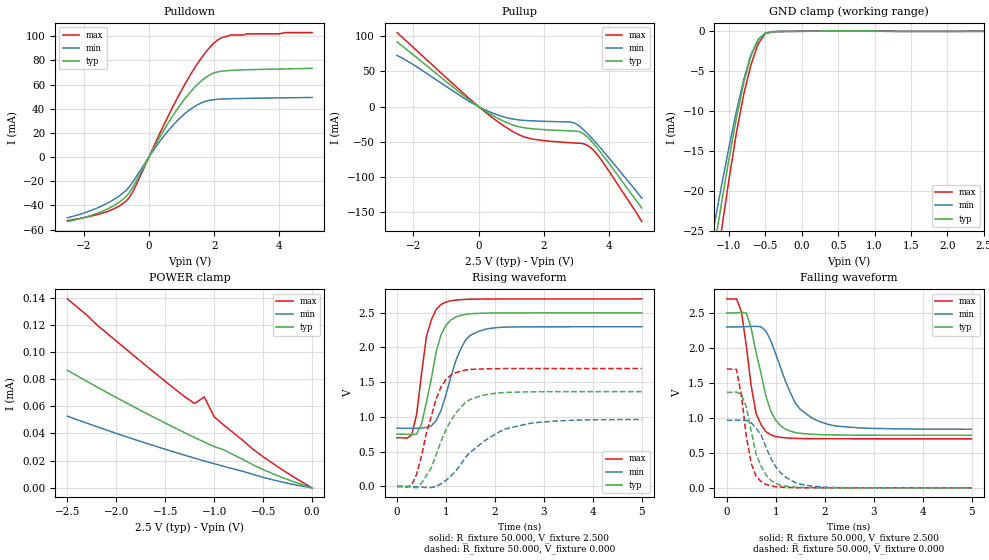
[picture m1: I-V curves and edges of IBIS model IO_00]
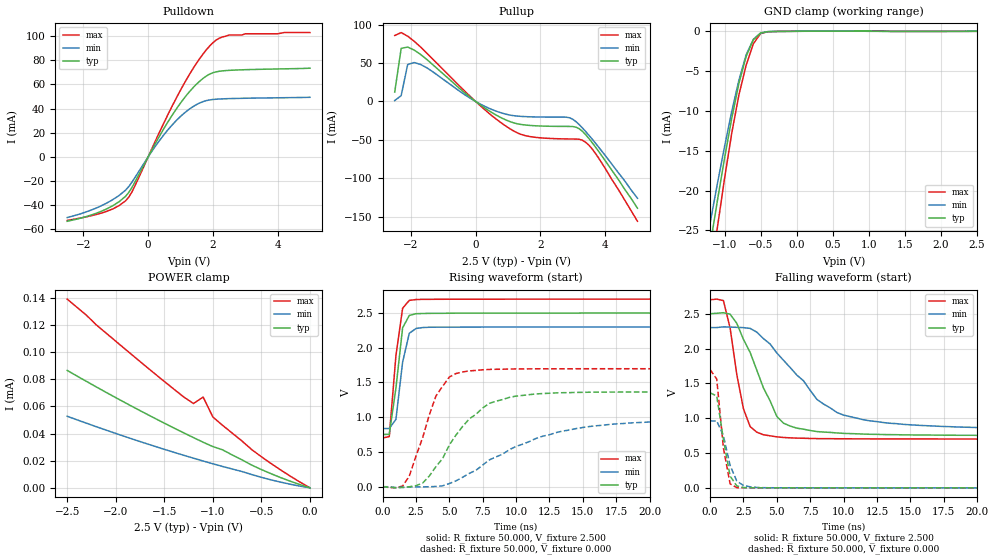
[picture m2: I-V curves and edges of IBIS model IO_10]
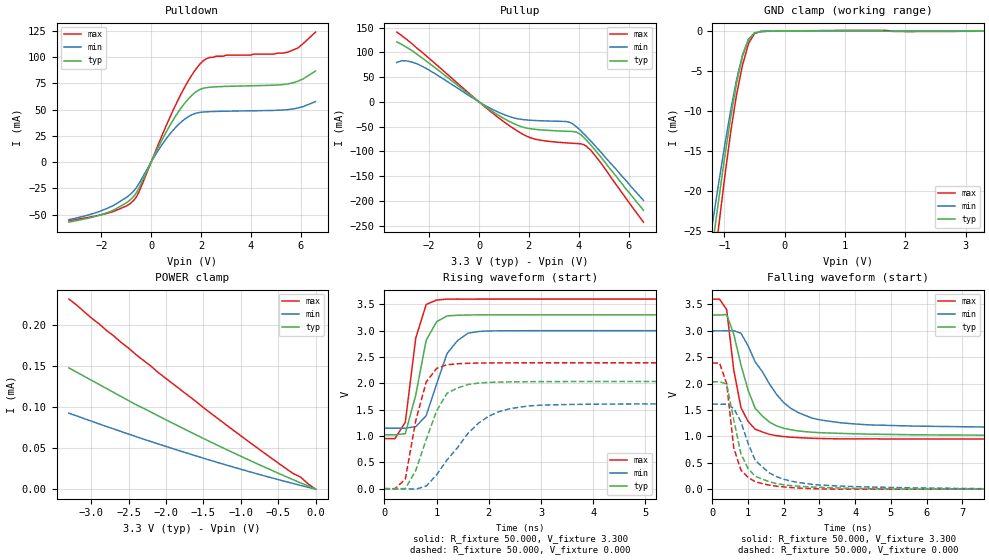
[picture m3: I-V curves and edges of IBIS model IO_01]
| / 7\'7   Xilinx XC9500XL I/O Buffer IBIS File
| \ \   Xilinx Inc.
| / /   2100 Logic Drive
| \_\/.\   San Jose,   CA 95124
[IBIS ver]   3.2
[File name]   trigger_a.ibs
[File Rev]   2.2
[Date]   Sat Aug 03 14:31:19 2002
[Source]   Spice netlist
[Notes]   - max/min process data included in this ibis model
   - Control flag setting:
   SLW=0 - fast slew rate
   SLW=1 - slow slew rate
   VIO=0 - 2.5V Vddio
   VIO=1 - 3.3V Vddio
   - Created by Joey Jia x4437
[Disclaimer] The data in this model is derived from SPICE simulations
   using modeling information extracted from the target pro-
   cess. While a great deal of care has been take to provide
   information that is accurate, this model is considered
   preliminary as it has not been verified by actual silicon
   measurement. Treat the data in this model as preliminary
   until actual silicon verification is performed.
[Copyright]   Xilinx Inc.
|   Component XC9500XL
|   >>> Make Your Selection of the Package type Below <<<
[Component]   XC9500XL
[Manufacturer]   Xilinx Inc.
[Package]
| variable   min   typ   max
R_pkg   0.079200   0.084800   0.090400
L_pkg   4.700nH   5.200nH   5.700nH
C_pkg   0.400pF   0.550pF   0.700pF
[Pin]  signal_name   model_name   R_pin   L_pin   C_pin
90   data<6>   IO_11
79   data<4>   IO_11
27   data<0>   IO_11
59   data<2>   IO_11
22   clock   IO_11
12   rd   IO_11
8   ctr_a1   IO_11
56   ctr_a0   IO_11
95   data<7>   IO_11
74   data<5>   IO_11
30   wr2   IO_11
99   wr0   IO_11
42   wr1   IO_11
91   ctr_data<3>   IO_11
85   ctr_data<5>   IO_11
92   ctr_data<7>   IO_11
1   ctr_data<1>   IO_11
23   ctr_data<2>   IO_11
3   ctr_data<4>   IO_11
77   ctr_data<6>   IO_11
94   data<3>   IO_11
89   ctr_data<0>   IO_11
18   data<1>   IO_11
13   addr<0>   IO_01
41   addr<10>   IO_01
87   addr<11>   IO_01
93   addr<12>   IO_01
96   addr<13>   IO_01
97   addr<14>   IO_01
14   addr<1>   IO_01
50   addr<2>   IO_01
53   addr<3>   IO_01
65   addr<4>   IO_01
37   addr<5>   IO_01
60   addr<6>   IO_01
61   addr<7>   IO_01
55   addr<8>   IO_01
64   addr<9>   IO_01
6   addr<15>   IO_01
28   clkout   IO_01
39   memrd   IO_01
11   ctlout<0>   IO_01
72   ctlout<1>   IO_01
76   ctlout<2>   IO_01
70   ctlout<3>   IO_01
86   ctlout<4>   IO_01
78   ctlout<5>   IO_01
82   ctlout<6>   IO_01
81   ctlout<7>   IO_01
10   go_out   IO_01
| Models and submodels in the file (4): IO_00 (I/O), IO_10 (I/O), IO_01 (I/O), IO_11 (I/O)
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|   Model IO_00
[Model]   IO_00
Model_type   I/O
Polarity   Inverting
Enable   Active-High
Vinl =   0.800V
Vinh =   2.000V
Vmeas =   1.250V
Cref =  50.000pF
Rref =   1.000M
Vref =  0.000V
C_comp   6.700pF   5.700pF   7.600pF
[Temperature Range]   50.000   100.000   0.000
[Voltage Range]   2.500V   2.300V   2.700V
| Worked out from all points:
|   slope of the pulldown table from 0 to 0.375 V, typ, clamps not added: 20.4 ohm
|   slope of the pullup table from 0 to 0.375 V, typ, clamps not added: 33.7 ohm
|   GND clamp passes 1 mA (typ) near -0.59 V on its own axis
|   rising waveform, R_fixture 50.000, V_fixture 2.500: 20-80 % time 320ps typ, 408ps min, 249ps max; typ from 0.752 V to 2.5 V
|   rising waveform, R_fixture 50.000, V_fixture 0.000: 20-80 % time 544ps typ, 897ps min, 394ps max; typ from 0 V to 1.36 V
|   falling waveform, R_fixture 50.000, V_fixture 2.500: 20-80 % time 361ps typ, 541ps min, 246ps max; typ from 2.5 V to 0.752 V
|   falling waveform, R_fixture 50.000, V_fixture 0.000: 20-80 % time 313ps typ, 452ps min, 216ps max; typ from 1.36 V to 0 V
[Pulldown]
| voltage   I(typ)   I(min)   I(max)
-2.5V     -53.3mA    -50.18mA   -52.6mA
-1.3V     -43.29mA   -38.5mA    -45.24mA
-900mV    -37.13mA   -31.98mA   -40.37mA
-600mV    -29.49mA   -24.58mA   -33.4mA
-400mV    -20.36mA   -16.75mA   -23.48mA
300mV     14.82mA    11.72mA    17.61mA
900mV     40.85mA    30.95mA    50.29mA
1.3V      54.75mA    40.1mA     69.38mA
1.6V      62.9mA     44.78mA    81.74mA
2.1V      70.47mA    47.8mA     96.78mA
2.5V      71.69mA    48.3mA     101mA
5V        73.49mA    49.4mA     103mA
[Pullup]
| voltage   I(typ)   I(min)   I(max)
-2.5V     91.64mA    72.63mA    105mA
-200mV    6.597mA    5.069mA    7.944mA
400mV     -11.81mA   -8.597mA   -14.94mA
900mV     -23.39mA   -16.16mA   -31.1mA
1.3V      -29.26mA   -19.18mA   -41.18mA
1.6V      -31.21mA   -20.09mA   -45.4mA
2.8V      -34.35mA   -21.93mA   -51.18mA
3V        -34.86mA   -24.83mA   -51.75mA
3.3V      -41.63mA   -36.61mA   -54.02mA
3.6V      -56.87mA   -51.52mA   -65.98mA
4V        -80.78mA   -73.13mA   -91.93mA
5V        -144mA     -130mA     -163mA
[GND_clamp]
| voltage   I(typ)   I(min)   I(max)
-2.5V     -106mA     -95.22mA   -120mA
-1.2V     -26.97mA   -24.12mA   -31.21mA
-1.1V     -21.35mA   -19.21mA   -24.73mA
-1V       -15.97mA   -14.5mA    -18.53mA
-900mV    -10.95mA   -10.08mA   -12.81mA
-800mV    -6.536mA   -6.124mA   -7.972mA
-700mV    -3.151mA   -2.957mA   -4.247mA
-600mV    -1.058mA   -1.006mA   -1.557mA
-500mV    -212uA     -231uA     -287uA
-400mV    -45.28uA   -47.34uA   -59.63uA
100mV     5.458uA    3.158uA    9.403uA
2.5V      1.486nA    2.623uA    -7.463uA
[POWER_clamp]
| voltage   I(typ)   I(min)   I(max)
-2.5V     86.5uA     52.74uA    139uA
-2.3V     78.34uA    47.57uA    127uA
-2.2V     74.33uA    45.03uA    120uA
-1.7V     55.02uA    32.94uA    90.07uA
-1.3V     40.51uA    23.99uA    66.94uA
-1.2V     37.02uA    21.86uA    62.11uA
-1.1V     33.6uA     19.77uA    66.85uA
-1V       30.39uA    17.73uA    52.18uA
-900mV    28uA       15.75uA    46.06uA
-500mV    13.46uA    7.741uA    22.89uA
-200mV    4.817uA    2.623uA    8.493uA
0V        1.483nA    6.217nA    302pA
[Ramp]
| variable   typ   min   max
dV/dt_r   0.819/0.540n   0.578/0.904n   1.019/0.360n
dV/dt_f   1.049/0.330n   0.877/0.563n   1.199/0.228n
R_load = 50.000
[Rising Waveform]
R_fixture = 50.000
V_fixture = 2.500
V_fixture_min = 2.300
V_fixture_max = 2.700
L_fixture = 0.000H
C_fixture = 0.000F
| time   V(typ)   V(min)   V(max)
0s        752mV      837mV      701mV
300ps     747mV      837mV      741mV
400ps     754mV      837mV      1.035V
500ps     897mV      840mV      1.618V
600ps     1.209V     849mV      2.156V
700ps     1.547V     872mV      2.396V
900ps     2.186V     1.096V     2.62V
1.3ns     2.462V     1.976V     2.689V
1.7ns     2.493V     2.241V     2.697V
5ns       2.499V     2.299V     2.7V
[Rising Waveform]
R_fixture = 50.000
V_fixture = 0.000
V_fixture_min = 0.000
V_fixture_max = 0.000
L_fixture = 0.000H
C_fixture = 0.000F
| time   V(typ)   V(min)   V(max)
0s        0V         0V         0V
300ps     -11.79mV   -884uV     20.59mV
500ps     44.89mV    -9.011mV   438mV
700ps     268mV      -16.52mV   1.007V
900ps     654mV      38.09mV    1.433V
1.2ns     1.053V     225mV      1.639V
1.5ns     1.254V     496mV      1.684V
2.2ns     1.353V     825mV      1.697V
3.2ns     1.364V     940mV      1.698V
5ns       1.365V     964mV      1.698V
[Falling Waveform]
R_fixture = 50.000
V_fixture = 2.500
V_fixture_min = 2.300
V_fixture_max = 2.700
L_fixture = 0.000H
C_fixture = 0.000F
| time   V(typ)   V(min)   V(max)
0s        2.5V       2.3V       2.7V
200ps     2.499V     2.299V     2.701V
300ps     2.509V     2.3V       2.52V
400ps     2.497V     2.304V     2.029V
500ps     2.278V     2.307V     1.454V
600ps     1.933V     2.309V     1.063V
900ps     1.097V     2.102V     758mV
1.4ns     790mV      1.212V     707mV
1.9ns     761mV      946mV      703mV
5ns       752mV      838mV      701mV
[Falling Waveform]
R_fixture = 50.000
V_fixture = 0.000
V_fixture_min = 0.000
V_fixture_max = 0.000
L_fixture = 0.000H
C_fixture = 0.000F
| time   V(typ)   V(min)   V(max)
0s        1.365V     965mV      1.698V
200ps     1.369V     967mV      1.693V
300ps     1.338V     970mV      1.318V
400ps     1.155V     963mV      737mV
500ps     810mV      930mV      350mV
600ps     480mV      854mV      165mV
800ps     186mV      587mV      48.87mV
1.1ns     37.06mV    216mV      10.58mV
1.5ns     6.726mV    52.91mV    1.766mV
5ns       9.319uV    61.34uV    0V
|   Model IO_10
[Model]   IO_10
Model_type   I/O
Polarity   Inverting
Enable   Active-High
Vinl =   0.800V
Vinh =   2.000V
Vmeas =   1.250V
Cref =  50.000pF
Rref =   1.000M
Vref =  0.000V
C_comp   6.700pF   5.700pF   7.600pF
[Temperature Range]   50.000   100.000   0.000
[Voltage Range]   2.500V   2.300V   2.700V
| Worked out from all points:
|   slope of the pulldown table from 0 to 0.375 V, typ, clamps not added: 20.4 ohm
|   slope of the pullup table from 0 to 0.375 V, typ, clamps not added: 33.7 ohm
|   GND clamp passes 1 mA (typ) near -0.59 V on its own axis
|   rising waveform, R_fixture 50.000, V_fixture 2.500: 20-80 % time 660ps typ, 660ps min, 641ps max; typ from 0.752 V to 2.5 V
|   rising waveform, R_fixture 50.000, V_fixture 0.000: 20-80 % time 3.33ns typ, 6.23ns min, 1.86ns max; typ from 0 V to 1.36 V
|   falling waveform, R_fixture 50.000, V_fixture 2.500: 20-80 % time 2.37ns typ, 4.34ns min, 1.07ns max; typ from 2.5 V to 0.753 V
|   falling waveform, R_fixture 50.000, V_fixture 0.000: 20-80 % time 719ps typ, 837ps min, 624ps max; typ from 1.36 V to 0 V
[Pulldown]
| voltage   I(typ)   I(min)   I(max)
-2.5V     -53.3mA    -50.18mA   -52.6mA
-1.3V     -43.29mA   -38.5mA    -45.24mA
-900mV    -37.13mA   -31.98mA   -40.37mA
-600mV    -29.49mA   -24.58mA   -33.4mA
-400mV    -20.36mA   -16.75mA   -23.48mA
300mV     14.82mA    11.72mA    17.61mA
900mV     40.85mA    30.95mA    50.29mA
1.3V      54.75mA    40.1mA     69.38mA
1.6V      62.9mA     44.78mA    81.74mA
2.1V      70.47mA    47.8mA     96.78mA
2.5V      71.69mA    48.3mA     101mA
5V        73.49mA    49.4mA     103mA
[Pullup]
| voltage   I(typ)   I(min)   I(max)
-2.5V     12.24mA    1.198mA    85.88mA
-2.3V     69.18mA    7.658mA    89.72mA
-2.1V     70.87mA    48.15mA    85.02mA
-1.9V     66.99mA    50.7mA     78.46mA
-1.7V     61.23mA    48.2mA     70.91mA
0V        380pA      458pA      152pA
1V        -25.2mA    -17.18mA   -33.92mA
1.6V      -30.91mA   -19.83mA   -45.07mA
2.9V      -32.48mA   -21.2mA    -48.83mA
3.2V      -35.52mA   -30.12mA   -49.19mA
3.6V      -53.59mA   -49.02mA   -61.75mA
5V        -139mA     -126mA     -156mA
[GND_clamp]
| voltage   I(typ)   I(min)   I(max)
-2.5V     -106mA     -95.22mA   -120mA
-1.2V     -26.97mA   -24.12mA   -31.21mA
-1.1V     -21.35mA   -19.21mA   -24.73mA
-1V       -15.97mA   -14.5mA    -18.53mA
-900mV    -10.95mA   -10.08mA   -12.81mA
-800mV    -6.536mA   -6.124mA   -7.972mA
-700mV    -3.151mA   -2.957mA   -4.247mA
-600mV    -1.058mA   -1.006mA   -1.557mA
-500mV    -212uA     -231uA     -287uA
-400mV    -45.28uA   -47.34uA   -59.63uA
100mV     5.458uA    3.158uA    9.403uA
2.5V      1.485nA    2.623uA    -7.463uA
[POWER_clamp]
| voltage   I(typ)   I(min)   I(max)
-2.5V     86.5uA     52.74uA    139uA
-2.3V     78.34uA    47.57uA    127uA
-2.2V     74.33uA    45.03uA    120uA
-1.7V     55.02uA    32.94uA    90.07uA
-1.3V     40.51uA    23.99uA    66.94uA
-1.2V     37.02uA    21.86uA    62.11uA
-1.1V     33.6uA     19.77uA    66.85uA
-1V       30.39uA    17.73uA    52.18uA
-900mV    28uA       15.75uA    46.06uA
-500mV    13.46uA    7.741uA    22.89uA
-200mV    4.817uA    2.623uA    8.493uA
0V        1.483nA    6.217nA    302pA
[Ramp]
| variable   typ   min   max
dV/dt_r   0.818/3.238n   0.571/6.157n   1.019/1.658n
dV/dt_f   1.048/2.140n   0.869/4.289n   1.199/1.164n
R_load = 50.000
[Rising Waveform]
R_fixture = 50.000
V_fixture = 2.500
V_fixture_min = 2.300
V_fixture_max = 2.700
L_fixture = 0.000H
C_fixture = 0.000F
| time   V(typ)   V(min)   V(max)
0s        752mV      837mV      701mV
500ps     753mV      837mV      721mV
1ns       1.42V      969mV      1.886V
1.5ns     2.287V     1.792V     2.568V
2ns       2.465V     2.208V     2.682V
2.5ns     2.49V      2.277V     2.694V
3.5ns     2.495V     2.295V     2.697V
25ns      2.5V       2.299V     2.7V
[Rising Waveform]
R_fixture = 50.000
V_fixture = 0.000
V_fixture_min = 0.000
V_fixture_max = 0.000
L_fixture = 0.000H
C_fixture = 0.000F
| time   V(typ)   V(min)   V(max)
0s        0V         0V         0V
1.5ns     -7.201mV   -12.08mV   9.131mV
2ns       -1.378mV   -4.713mV   151mV
3ns       51.72mV    -2.604mV   704mV
4ns       290mV      3.048mV    1.307V
5.5ns     744mV      84.1mV     1.629V
8ns       1.2V       386mV      1.688V
10ns      1.304V     580mV      1.695V
15.5ns    1.36V      866mV      1.698V
25ns      1.364V     952mV      1.698V
[Falling Waveform]
R_fixture = 50.000
V_fixture = 2.500
V_fixture_min = 2.300
V_fixture_max = 2.700
L_fixture = 0.000H
C_fixture = 0.000F
| time   V(typ)   V(min)   V(max)
0s        2.5V       2.3V       2.7V
1ns       2.514V     2.311V     2.688V
1.5ns     2.493V     2.308V     2.294V
2.5ns     2.131V     2.3V       1.134V
3.5ns     1.689V     2.235V     799mV
5ns       1.024V     1.936V     732mV
5.5ns     928mV      1.831V     723mV
8ns       808mV      1.27V      707mV
10ns      782mV      1.044V     704mV
25ns      753mV      851mV      701mV
[Falling Waveform]
R_fixture = 50.000
V_fixture = 0.000
V_fixture_min = 0.000
V_fixture_max = 0.000
L_fixture = 0.000H
C_fixture = 0.000F
| time   V(typ)   V(min)   V(max)
0s        1.364V     960mV      1.698V
500ps     1.318V     961mV      1.56V
1ns       694mV      747mV      571mV
1.5ns     169mV      321mV      59.13mV
2ns       27.93mV    97.21mV    2.6mV
2.5ns     4.716mV    34.55mV    1.839mV
3ns       2.075mV    15.5mV     1.398mV
4ns       1.283mV    2.462mV    1.078mV
25ns      21.8uV     99uV       65nV
|   Model IO_01
[Model]   IO_01
Model_type   I/O
Polarity   Inverting
Enable   Active-High
Vinl =   0.800V
Vinh =   2.000V
Vmeas =   1.650V
Cref =  50.000pF
Rref =   1.000M
Vref =  0.000V
C_comp   6.700pF   5.700pF   7.600pF
[Temperature Range]   50.000   100.000   0.000
[Voltage Range]   3.300V   3.000V   3.600V
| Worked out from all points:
|   slope of the pulldown table from 0 to 0.495 V, typ, clamps not added: 20.7 ohm
|   slope of the pullup table from 0 to 0.495 V, typ, clamps not added: 27.8 ohm
|   GND clamp passes 1 mA (typ) near -0.59 V on its own axis
|   rising waveform, R_fixture 50.000, V_fixture 3.300: 20-80 % time 297ps typ, 408ps min, 239ps max; typ from 1.02 V to 3.3 V
|   rising waveform, R_fixture 50.000, V_fixture 0.000: 20-80 % time 469ps typ, 827ps min, 316ps max; typ from 0 V to 2.04 V
|   falling waveform, R_fixture 50.000, V_fixture 3.300: 20-80 % time 642ps typ, 1.14ns min, 392ps max; typ from 3.3 V to 1.02 V
|   falling waveform, R_fixture 50.000, V_fixture 0.000: 20-80 % time 482ps typ, 780ps min, 329ps max; typ from 2.04 V to 0 V
[Pulldown]
| voltage   I(typ)   I(min)   I(max)
-3.3V     -57.2mA    -54.8mA    -55.7mA
-1.7V     -47.57mA   -43.39mA   -48.32mA
-700mV    -32.66mA   -27.57mA   -36.39mA
-500mV    -25.26mA   -20.88mA   -29mA
300mV     14.82mA    11.72mA    17.61mA
900mV     40.85mA    30.95mA    50.29mA
1.6V      62.9mA     44.78mA    81.73mA
2.1V      70.46mA    47.8mA     96.79mA
3V        72.23mA    48.59mA    102mA
5.5V      74.68mA    50.15mA    105mA
5.9V      77.27mA    51.71mA    109mA
6.6V      86.93mA    57.76mA    124mA
[Pullup]
| voltage   I(typ)   I(min)   I(max)
-3.3V     121mA      79.65mA    141mA
-2.9V     110mA      82.69mA    126mA
-2.3V     89.33mA    72.44mA    101mA
300mV     -11.04mA   -8.824mA   -12.73mA
1.5V      -46.27mA   -33.63mA   -57.51mA
1.9V      -52.76mA   -36.44mA   -68.97mA
2.3V      -55.67mA   -37.72mA   -75.79mA
3.7V      -59.69mA   -42.64mA   -83.42mA
4V        -63.32mA   -54.46mA   -84.35mA
4.2V      -71.44mA   -64.25mA   -86.4mA
4.5V      -87.94mA   -80.06mA   -98.42mA
6.6V      -219mA     -199mA     -243mA
[GND_clamp]
| voltage   I(typ)   I(min)   I(max)
-3.3V     -155mA     -140mA     -172mA
-1.2V     -26.97mA   -24.12mA   -31.21mA
-1.1V     -21.35mA   -19.21mA   -24.73mA
-1V       -15.97mA   -14.5mA    -18.53mA
-900mV    -10.95mA   -10.08mA   -12.81mA
-800mV    -6.54mA    -6.125mA   -7.981mA
-700mV    -3.156mA   -2.96mA    -4.255mA
-600mV    -1.062mA   -1.009mA   -1.564mA
-500mV    -216uA     -233uA     -293uA
-400mV    -48.58uA   -49.49uA   -64.66uA
700mV     37.32uA    20.73uA    65.45uA
3.3V      1.628nA    6.9uA      -17.62uA
[POWER_clamp]
| voltage   I(typ)   I(min)   I(max)
-3.3V     148uA      92.8uA     232uA
-2.4V     103uA      64.12uA    164uA
-1.5V     61.88uA    37.81uA    99.54uA
-500mV    19.51uA    11.69uA    31.91uA
-300mV    11.57uA    6.9uA      19.07uA
-200mV    7.689uA    4.565uA    14.73uA
-100mV    4uA        2.274uA    6.481uA
0V        1.628nA    6.511nA    380pA
[Ramp]
| variable   typ   min   max
dV/dt_r   1.221/0.443n   0.967/0.760n   1.433/0.321n
dV/dt_f   1.366/0.616n   1.101/1.088n   1.589/0.410n
R_load = 50.000
[Rising Waveform]
R_fixture = 50.000
V_fixture = 3.300
V_fixture_min = 3.000
V_fixture_max = 3.600
L_fixture = 0.000H
C_fixture = 0.000F
| time   V(typ)   V(min)   V(max)
0s        1.023V     1.148V     951mV
200ps     1.023V     1.148V     949mV
400ps     1.044V     1.148V     1.262V
600ps     1.779V     1.178V     2.859V
800ps     2.818V     1.386V     3.496V
1ns       3.169V     1.985V     3.581V
1.2ns     3.279V     2.566V     3.598V
1.6ns     3.297V     2.951V     3.598V
1.8ns     3.299V     2.983V     3.599V
10ns      3.299V     3V         3.599V
[Rising Waveform]
R_fixture = 50.000
V_fixture = 0.000
V_fixture_min = 0.000
V_fixture_max = 0.000
L_fixture = 0.000H
C_fixture = 0.000F
| time   V(typ)   V(min)   V(max)
0s        0V         0V         0V
200ps     -298uV     110uV      -3.088mV
400ps     1.188mV    -1.293mV   181mV
600ps     345mV      -9.507mV   1.291V
800ps     933mV      48.75mV    2.024V
1ns       1.477V     263mV      2.284V
1.2ns     1.811V     546mV      2.353V
1.8ns     2.004V     1.242V     2.385V
2.6ns     2.029V     1.549V     2.389V
10ns      2.035V     1.611V     2.389V
[Falling Waveform]
R_fixture = 50.000
V_fixture = 3.300
V_fixture_min = 3.000
V_fixture_max = 3.600
L_fixture = 0.000H
C_fixture = 0.000F
| time   V(typ)   V(min)   V(max)
0s        3.3V       3V         3.6V
200ps     3.299V     2.999V     3.602V
400ps     3.309V     3.001V     3.403V
600ps     2.934V     3.003V     2.257V
800ps     2.357V     2.955V     1.547V
1.2ns     1.532V     2.409V     1.136V
1.6ns     1.27V      1.992V     1.039V
2ns       1.154V     1.638V     997mV
3ns       1.071V     1.314V     960mV
10ns      1.023V     1.165V     951mV
[Falling Waveform]
R_fixture = 50.000
V_fixture = 0.000
V_fixture_min = 0.000
V_fixture_max = 0.000
L_fixture = 0.000H
C_fixture = 0.000F
| time   V(typ)   V(min)   V(max)
0s        2.035V     1.611V     2.389V
200ps     2.036V     1.611V     2.391V
400ps     1.992V     1.61V      2.003V
600ps     1.311V     1.528V     779mV
800ps     669mV      1.276V     362mV
1ns       391mV      871mV      223mV
1.2ns     244mV      546mV      141mV
1.8ns     105mV      236mV      56.13mV
2.8ns     40.08mV    90.65mV    9.067mV
10ns      30.04uV    1.855mV    -12.44uV
